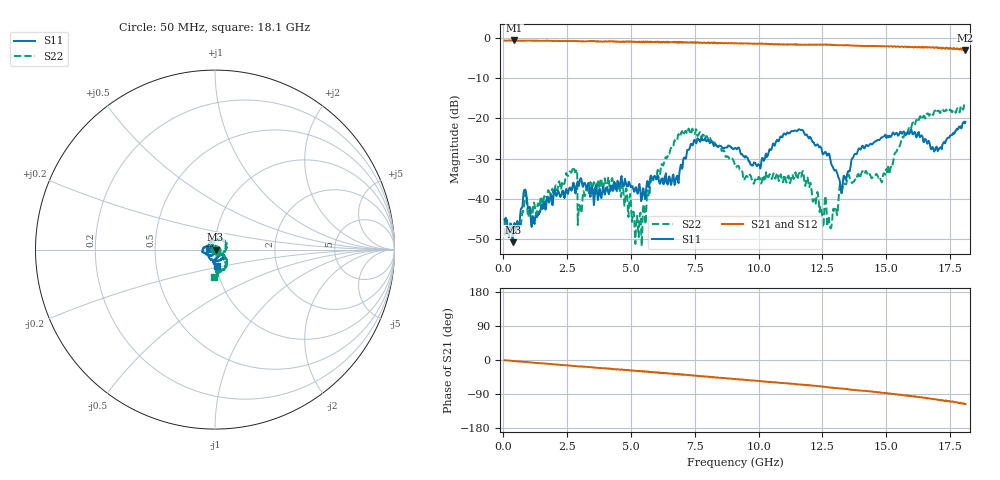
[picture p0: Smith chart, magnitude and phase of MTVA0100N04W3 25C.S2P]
! Network Analyzer HP8720D.06.14 Serial No. US36140669
! 17 Jan 2005  10:24:46
! Frequency  S11  S21  S12  S22
# HZ  S  DB R 50
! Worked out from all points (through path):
!   801 points, 50 MHz to 18.1 GHz, reference 50 ohm
!   highest |S21| = -0.72 dB at 433.6 MHz (marker M1); lowest = -3.2 dB at 18.1 GHz (marker M2)
!   group delay of S21, straight-line fit = 16.8 ps
!   lowest |S11| = -50.8 dB at 365.9 MHz (marker M3), VSWR 1.01, Z = 50.3 + j0.0478 ohm
!   |S11| at or under -10 dB: start of sweep to end of sweep
!   |S22| runs from -51.7 to -16.3 dB; largest |S21 - S12| = 0.028
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5e7  -45.15 -52.8  -0.74 -0.8  -0.76 -1.1  -49.11 -24.6
3.65875e8  -50.81 9.5  -0.73 -2.7  -0.74 -2.9  -49.63 -18.4
4.335625e8  -46.00 24.1  -0.72 -2.9  -0.74 -3.2  -45.69 -2.7
8.396875e8  -37.79 26.1  -0.78 -4.8  -0.81 -5.2  -40.37 -78.9
1.178125e9  -44.86 21.1  -0.77 -7.3  -0.78 -7.4  -41.41 144.2
2.689812e9  -37.74 64.1  -0.83 -15.2  -0.85 -15.6  -33.12 121.4
3.073375e9  -35.79 78.8  -0.91 -17.3  -0.89 -17.5  -42.93 -143.8
4.336875e9  -35.75 48.8  -0.98 -24.0  -0.96 -24.2  -38.09 148.8
5.352188e9  -37.48 124.7  -1.02 -30.0  -1.04 -30.0  -43.59 152.5
6.074188e9  -34.44 -155.2  -1.18 -34.0  -1.17 -34.1  -33.11 136.5
6.796188e9  -34.35 -174.3  -1.27 -37.6  -1.23 -37.6  -25.70 83.1
7.202312e9  -27.89 115.2  -1.12 -39.7  -1.19 -40.2  -23.89 45.2
9.075e9  -27.44 -171.7  -1.47 -50.2  -1.42 -50.4  -31.70 -75.5
1.000006e10  -31.40 -176.8  -1.54 -55.5  -1.54 -55.6  -34.58 -71.7
1.10605e10  -24.12 170.0  -1.74 -61.3  -1.75 -61.7  -35.42 -102.6
1.209838e10  -25.66 -147.9  -1.72 -67.6  -1.76 -67.8  -39.43 142.8
1.277525e10  -28.98 -113.1  -1.76 -72.6  -1.74 -72.7  -46.82 84.3
1.32265e10  -37.93 -123.4  -1.89 -75.2  -1.90 -75.4  -36.51 10.2
1.509919e10  -24.68 -103.5  -2.26 -88.5  -2.16 -88.9  -33.66 -54.0
1.624988e10  -23.54 -36.3  -2.40 -96.9  -2.40 -97.8  -20.96 -49.0
1.708469e10  -27.44 -60.0  -2.57 -105.8  -2.44 -106.3  -18.47 -73.2
1.81e10  -20.94 -83.6  -3.15 -116.5  -3.03 -117.0  -16.41 -91.8
